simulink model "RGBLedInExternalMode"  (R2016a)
settings: Solver=FixedStepAuto  StartTime=0.0  StopTime=Inf  RelTol=1e-3
PreLoadFcn:
  | R = Simulink.Parameter;
  | G = Simulink.Parameter;
  | B = Simulink.Parameter;
libraries: miniQ x1

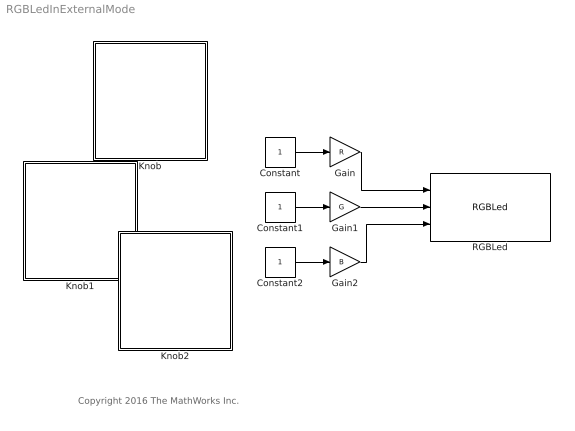
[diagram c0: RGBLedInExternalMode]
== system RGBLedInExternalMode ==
  note: Copyright 2016 The MathWorks Inc.
  Constant : Constant
  Constant1 : Constant
  Constant2 : Constant
  Gain : Gain  Gain=R
  Gain1 : Gain  Gain=G
  Gain2 : Gain  Gain=B
  Knob : Subsystem  DialogController=hmiCreateDDGDialog  IsWebBlock=on
  Knob1 : Subsystem  DialogController=hmiCreateDDGDialog  IsWebBlock=on
  Knob2 : Subsystem  DialogController=hmiCreateDDGDialog  IsWebBlock=on
  RGBLed : miniQ/RGBLed
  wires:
  Constant/1 -> Gain/1
  Gain/1 -> RGBLed/1
  Constant1/1 -> Gain1/1
  Constant2/1 -> Gain2/1
  Gain1/1 -> RGBLed/2
  Gain2/1 -> RGBLed/3

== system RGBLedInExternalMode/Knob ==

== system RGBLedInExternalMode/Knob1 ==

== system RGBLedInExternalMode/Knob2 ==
